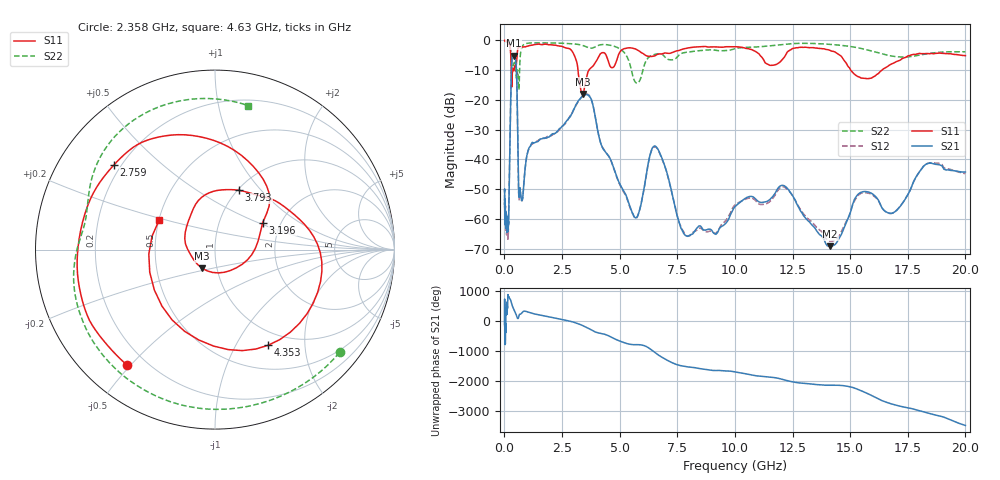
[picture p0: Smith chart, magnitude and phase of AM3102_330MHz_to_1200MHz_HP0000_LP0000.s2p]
! Date/Time: Tue, Sep 11, 2018 5:08 PM
! Network Analyzer: Agilent Technologies E8362B Rev: A.07.50.63
! Sweep from 0.010 to 20.000 GHz, 1601 Points, Sweep Type: LOG
! Power Supply: 4.950 V, 0.000 A
# Hz S DB R 50
!freq MagS11 AngS11 MagS21 AngS21 MagS12 AngS12 MagS22 AngS22
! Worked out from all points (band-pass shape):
!   1601 points, 10 MHz to 20 GHz, reference 50 ohm
!   highest |S21| = -5.17 dB at 399 MHz (marker M1); lowest = -69.2 dB at 14.14 GHz (marker M2)
!   |S21| within 3 dB of the highest: 314 MHz to 510.6 MHz (196.6 MHz wide, 47.7 % of centre)
!   lowest |S11| = -18.0 dB at 3.4 GHz (marker M3), VSWR 1.29, Z = 42.5 - j8.96 ohm
!   |S11| at or under -10 dB: 295 MHz to 351.7 MHz (56.7 MHz wide, 17.5 % of centre); 3.193 GHz to 3.664 GHz (471.5 MHz wide, 13.8 % of centre); 15.03 GHz to 16.38 GHz (1.351 GHz wide, 8.6 % of centre)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
!   |S22| runs from -16.6 to -0.2 dB; largest |S21 - S12| = 0.0069
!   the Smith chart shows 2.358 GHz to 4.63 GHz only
!   S11 on the Smith chart (normalised r, x): 2.358 GHz: 0.13, -0.49; 2.759 GHz: 0.17, +0.35; 3.196 GHz: 1.61, +0.54; 3.793 GHz: 1.02, +0.77; 4.353 GHz: 0.81, -1.37; 4.63 GHz: 0.50, +0.19
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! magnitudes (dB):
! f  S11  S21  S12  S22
! 10 MHz  0.0  -50.6  -50.7  -0.3
! 35.55 MHz  0.0  -61.0  -60.3  -0.3
! 126.4 MHz  -0.4  -62.3  -61.8  -0.7
! 173.8 MHz  -0.9  -61.4  -63.6  -1.1
! 399 MHz  -10.2  -5.2  -5.2  -8.1
! 447.2 MHz  -8.7  -5.7  -5.8  -7.4
! 530.6 MHz  -7.0  -11.5  -11.5  -12.5
! 635.6 MHz  -2.2  -52.8  -53.5  -15.9
! 1.59 GHz  -1.4  -33.1  -33.1  -0.8
! 2.358 GHz  -1.8  -29.9  -30.2  -0.9
! 2.759 GHz  -2.7  -26.6  -26.6  -1.0
! 3.196 GHz  -10.3  -20.4  -20.6  -1.3
! 3.4 GHz  -18.0  -18.5  -18.7  -1.7
! 3.793 GHz  -9.0  -20.4  -20.3  -2.6
! 4.353 GHz  -4.3  -37.2  -37.1  -1.4
! 4.63 GHz  -9.1  -40.4  -40.5  -1.7
! 5.652 GHz  -2.8  -59.4  -59.6  -13.7
! 6.58 GHz  -4.9  -35.7  -35.9  -4.6
! 7.882 GHz  -2.7  -65.7  -65.6  -4.0
! 12.09 GHz  -6.1  -48.7  -49.2  -1.3
! 14.14 GHz  -3.4  -69.2  -67.5  -1.3
! 20 GHz  -5.1  -44.2  -44.8  -3.8
